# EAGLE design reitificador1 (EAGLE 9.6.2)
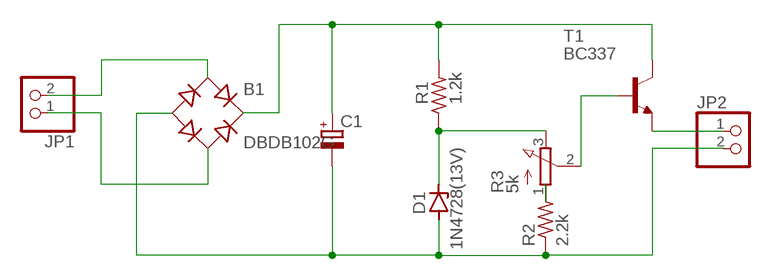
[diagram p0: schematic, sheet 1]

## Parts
B1  DBDB102G  [DB]
C1  CPOL-EUE5-8.5  [E5-8,5]
D1  1N4728(13V)  1N4728  [DO41Z10]
JP1  PINHD-1X2  [1X02]
JP2  PINHD-1X2  [1X02]
R1  1.2k  R-US_0204/7  [0204/7]
R2  2.2k  R-US_0204/7  [0204/7]
R3  5k  3RP/1610N  [3RP/1610N]
T1  BC337  [TO92]

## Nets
N$1: R2.2 R3.1(A)
N$2: B1.- C1.- D1.A JP2.2 R2.1
N$3: B1.AC1 JP1.2
N$4: JP2.1 T1.1(E)
N$5: B1.+ C1.+ R1.2 T1.3(C)
N$6: D1.C R1.1 R3.3(E)
N$7: R3.2(S) T1.2(B)
N$8: B1.AC2 JP1.1

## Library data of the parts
B1 = rectifier:DB?*G: Single Phase 1.0 AMP Glass Passivated Bridge Rectifier Taiwan Semiconductor Co.,Ltd. - TSC Source: http://www.taiwansemi.com/TSCbig5/ezcatfiles/cust/img/img/db101g.pdf http://www.ts.com.tw/db/pictures/modules/PDT/PDT060207001/DBLS201G.pdf
C1 = rcl:CPOL-EU: POLARIZED CAPACITOR, European symbol; SPICEPREFIX: C
D1 = diode:1N4728: Z DIODE
JP1 JP2 = pinhead:PINHD-1X2: PIN HEADER
R1 R2 = rcl:R-US_: RESISTOR, American symbol; SPICEPREFIX: R
R3 = pot:3RP/1610N: 16mm Potentiometer one level Source: http://www.alphapotentiometers.net/html/16mm_pot_2.html
T1 = transistor:BC337: NPN TRANSISTOR

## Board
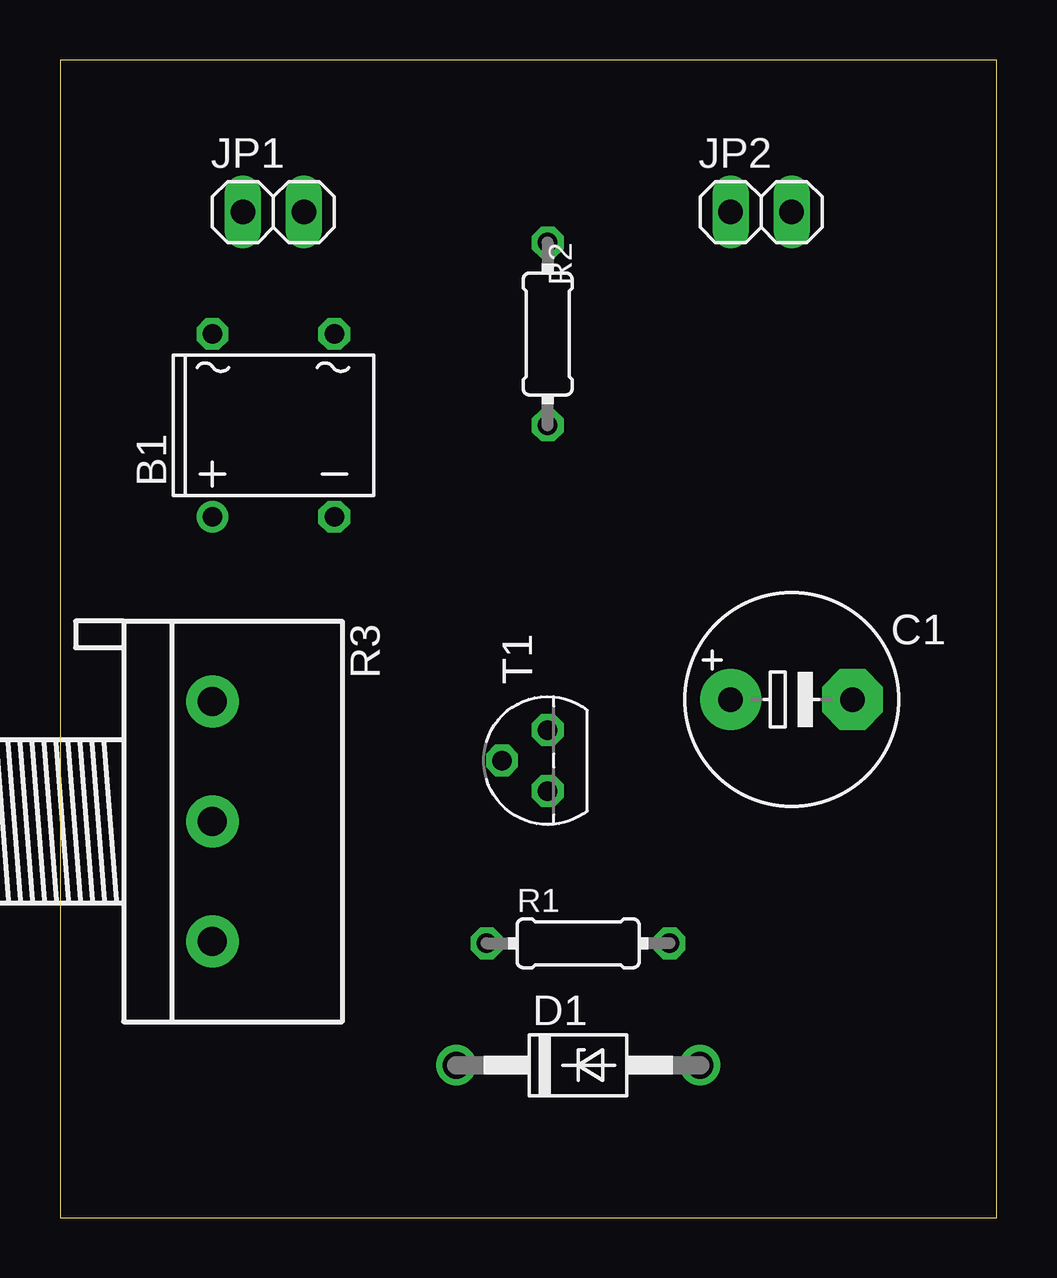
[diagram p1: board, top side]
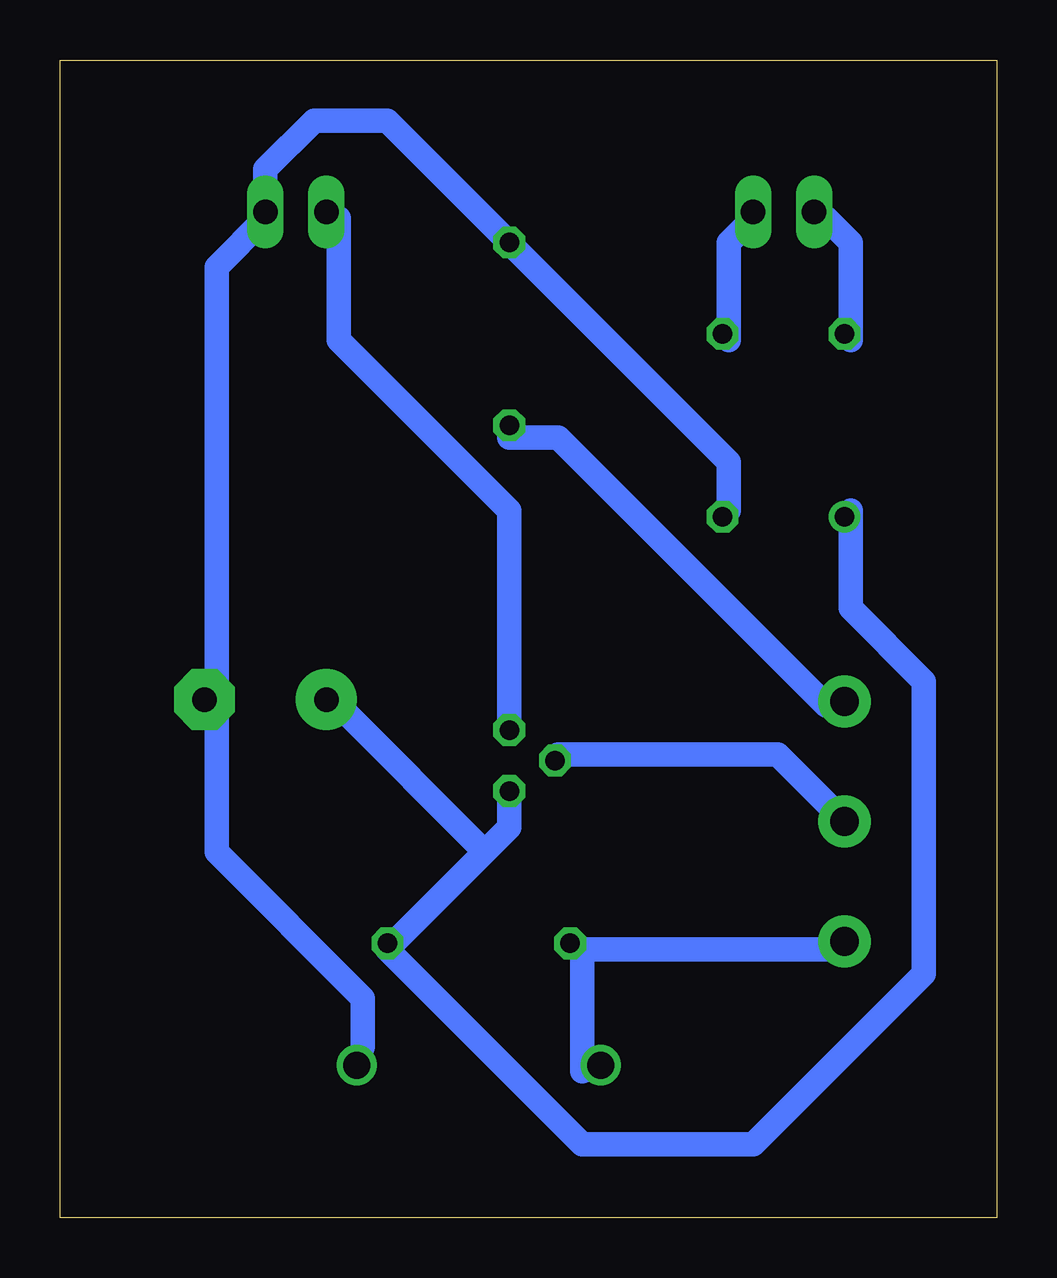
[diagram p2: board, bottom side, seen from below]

Size 39.04 x 48.25 mm. Coordinates in mm from the lower left corner, seen from the top.
Outline: 0,0 39.04,0 39.04,48.25 0,48.25 0,0
Copper layers (1*16): Top 0.035mm / dielectric 1.5mm / Bottom 0.035mm
Design rules "default *": minimum track width 40mil, minimum drill 0.35mm, track to track 40mil, track to pad 40mil, pad to pad 40mil, via to via 40mil, smd to smd 6mil, copper to edge 40mil, drill to drill 6mil, minimum pad ring 10mil, minimum via ring 8mil, stop-mask expansion 4mil, vias tented up to drill 0mil, thermal gap 10mil

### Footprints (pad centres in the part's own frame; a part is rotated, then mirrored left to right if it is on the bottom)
DB = drill 0.813: + -2.54,-3.81 | drill 0.813 octagon: - 2.54,-3.81; AC1 2.54,3.81; AC2 -2.54,3.81
E5-8,5 = drill 1.016 pad 2.54: + -2.54,0 | drill 1.016 pad 2.54 octagon: - 2.54,0
DO41Z10 = drill 1.118: A 5.08,0; C -5.08,0
1X02 = drill 1.016 long: 1 -1.27,0; 2 1.27,0
0204/7 = drill 0.813 octagon: 1 -3.81,0; 2 3.81,0
3RP/1610N = drill 1.2 pad 2.184: 1 -5,0; 2 0,0; 3 5,0
TO92 = drill 0.813 octagon: 1 1.27,0; 2 0,1.905; 3 -1.27,0

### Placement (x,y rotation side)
B1  8.89,33.02 0 top
C1  30.48,21.59 0 top
D1  21.59,6.35 0 top
JP1  8.89,41.91 0 top
JP2  29.21,41.91 0 top
R1  21.59,11.43 0 top
R2  20.32,36.83 270 top
R3  6.35,16.51 270 top
T1  20.32,19.05 90 top

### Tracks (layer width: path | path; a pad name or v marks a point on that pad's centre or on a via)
N$1
  Bottom 1.016: R2.2 20.32,32.51 18.29,32.51 7.11,21.34 R3.1
N$2
  Bottom 1.016: D1.A 26.42,7.11 26.42,9.14 32.51,15.24 32.51,21.34 C1.- 32.51,22.35 32.51,39.62 30.48,41.66 JP2.2 30.48,43.69 28.45,45.72 25.4,45.72 R2.1 11.18,31.5 11.18,29.46 B1.-
N$3
  Bottom 1.016: B1.AC1 11.18,36.58 11.18,40.64 10.16,41.66 JP1.2
N$4
  Bottom 1.016: T1.1 20.32,29.46 27.43,36.58 27.43,41.66 JP2.1
N$5
  Bottom 1.016: 21.34,15.24 20.32,16.26 T1.3 | 21.34,15.24 25.4,11.18 | 25.4,11.18 17.27,3.05 10.16,3.05 3.05,10.16 3.05,22.35 6.1,25.4 6.1,29.46 B1.+ | 25.4,11.18 R1.2 | 21.34,15.24 27.43,21.34 C1.+
N$6
  Bottom 1.016: 17.27,11.18 17.27,6.1 D1.C | 17.27,11.18 7.11,11.18 R3.3 | 17.27,11.18 R1.1
N$7
  Bottom 1.016: R3.2 9.14,19.3 18.29,19.3 T1.2
N$8
  Bottom 1.016: B1.AC2 6.1,36.58 6.1,40.64 7.11,41.66 JP1.1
